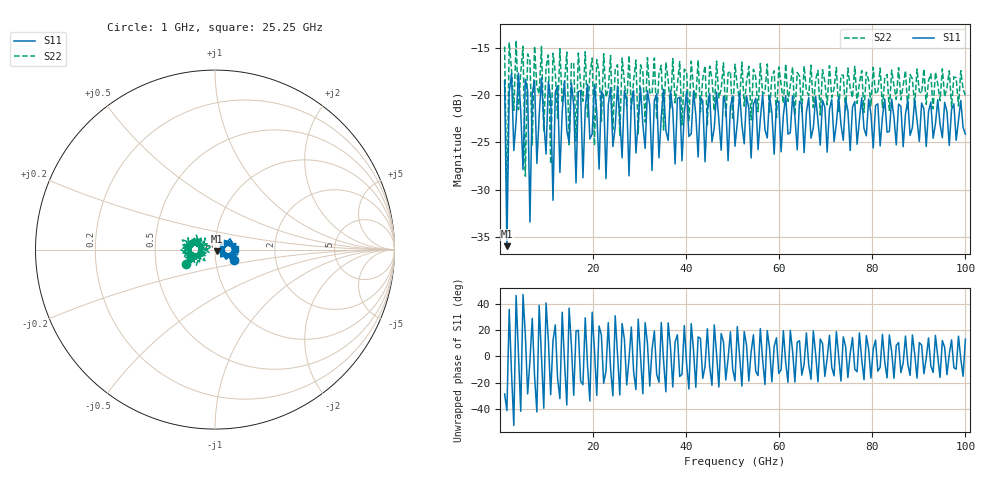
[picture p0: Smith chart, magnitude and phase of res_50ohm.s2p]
!Created with skrf (http://scikit-rf.org).
# GHz S RI R 50.0
!freq ReS11 ImS11 ReS21 ImS21 ReS12 ImS12 ReS22 ImS22
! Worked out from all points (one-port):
!   201 points, 1 GHz to 100 GHz, reference 50 ohm
!   lowest |S11| = -36.0 dB at 1.495 GHz (marker M1), VSWR 1.03, Z = 51.2 - j1.07 ohm
!   |S11| at or under -10 dB: start of sweep to end of sweep
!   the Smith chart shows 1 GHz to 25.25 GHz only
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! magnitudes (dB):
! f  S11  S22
! 1 GHz  -18.5  -14.9
! 1.495 GHz  -36.0  -31.6
! 1.99 GHz  -19.7  -14.4
! 2.485 GHz  -17.7  -17.3
! 4.96 GHz  -27.9  -14.9
! 5.455 GHz  -18.4  -28.6
! 6.445 GHz  -33.4  -16.4
! 6.94 GHz  -19.8  -25.3
! 7.435 GHz  -18.5  -14.8
! 7.93 GHz  -27.2  -19.2
! 10.4 GHz  -18.6  -15.8
! 10.9 GHz  -20.4  -27.3
! 11.39 GHz  -31.1  -15.6
! 12.38 GHz  -19.0  -22.5
! 17.34 GHz  -19.6  -18.9
! 17.83 GHz  -28.7  -20.7
! 18.82 GHz  -18.9  -22.4
! 34.16 GHz  -26.6  -17.8
! 50.5 GHz  -25.4  -16.8
! 67.33 GHz  -23.5  -21.3
! 83.67 GHz  -23.9  -21.6
! 100 GHz  -24.1  -20.0
